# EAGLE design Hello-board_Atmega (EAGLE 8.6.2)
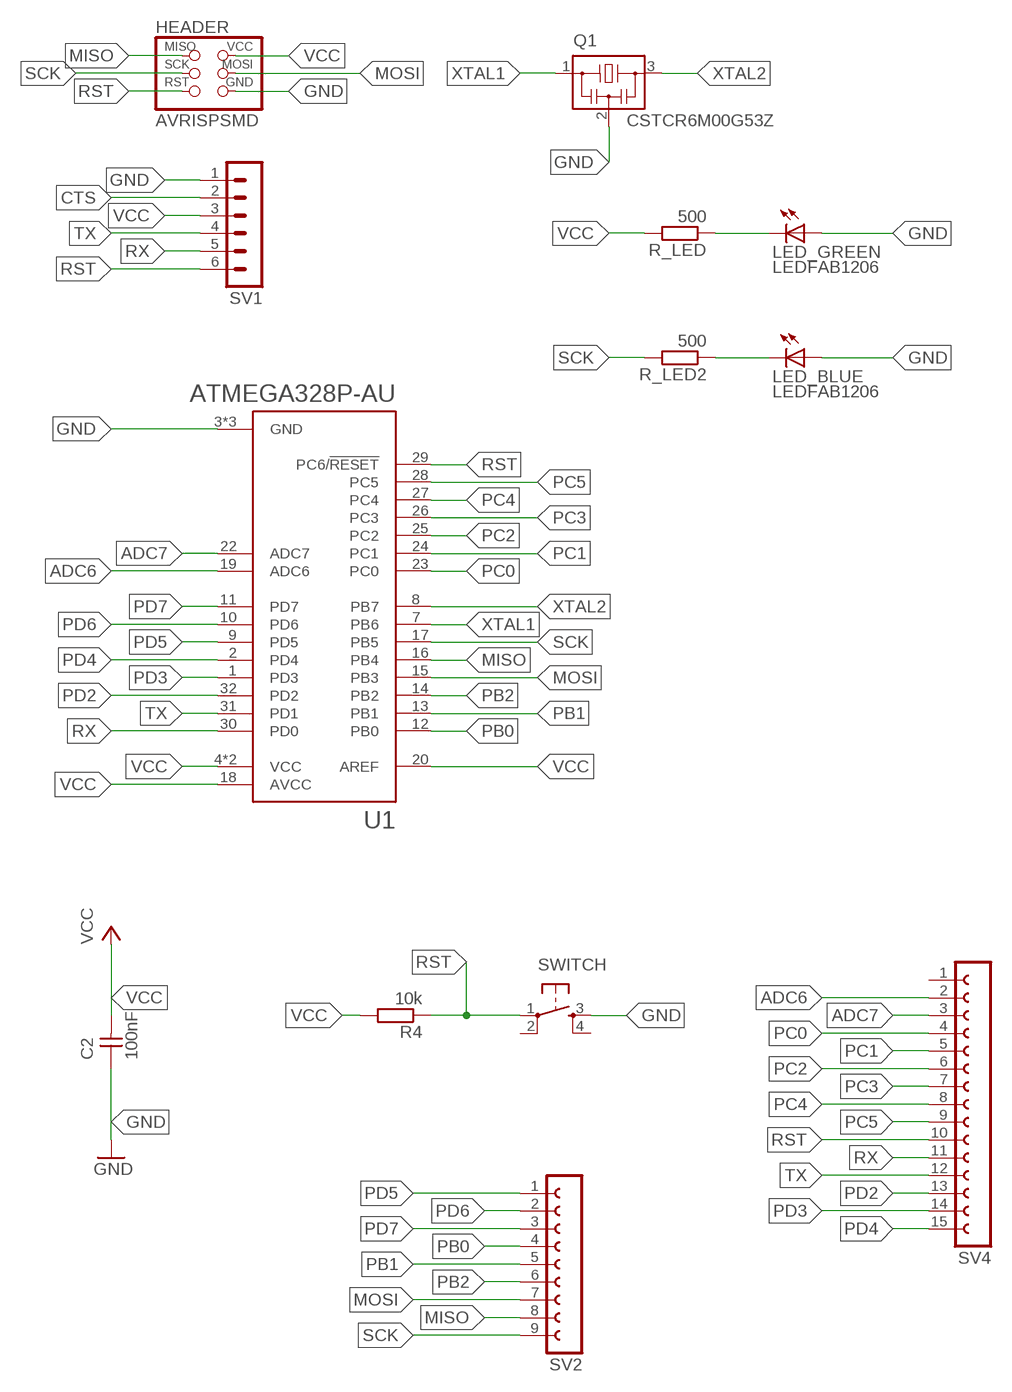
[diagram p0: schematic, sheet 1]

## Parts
C2  100nF  CAP-UNPOLARIZEDFAB  [C1206FAB]
HEADER  AVRISPSMD  [2X03SMD]
LED_BLUE  LEDFAB1206  [LED1206FAB]
LED_GREEN  LEDFAB1206  [LED1206FAB]
Q1  CSTCR6M00G53Z  [CSTCR6M]
R4  10k  R-EU_R1206  [R1206]
R_LED  500  R-EU_R1206  [R1206]
R_LED2  500  R-EU_R1206  [R1206]
SV1  MA06-1  [MA06-1]
SV2  FE09-1  [FE09]
SV4  FE15-1  [FE15]
SWITCH  6MM_SWITCH6MM_SWITCH  [6MM_SWITCH]
U1  ATMEGA328P-AU  [QFP80P900X900X120-32N]

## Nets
ADC6: SV4.2 U1.19(ADC6)
ADC7: SV4.3 U1.22(ADC7)
CTS: SV1.2
GND: C2.1 HEADER.6(GND) LED_BLUE.1(A) LED_GREEN.1(A) Q1.2 SV1.1 SWITCH.3(S) U1.3(GND) U1.5(GND) U1.21(GND)
MISO: HEADER.1(MISO) SV2.8 U1.16(PB4)
MOSI: HEADER.4(MOSI) SV2.7 U1.15(PB3)
N$21: LED_GREEN.2(C) R_LED.1
N$22: LED_BLUE.2(C) R_LED2.1
PB0: SV2.4 U1.12(PB0)
PB1: SV2.5 U1.13(PB1)
PB2: SV2.6 U1.14(PB2)
PC0: SV4.4 U1.23(PC0)
PC1: SV4.5 U1.24(PC1)
PC2: SV4.6 U1.25(PC2)
PC3: SV4.7 U1.26(PC3)
PC4: SV4.8 U1.27(PC4)
PC5: SV4.9 U1.28(PC5)
PD2: SV4.13 U1.32(PD2)
PD3: SV4.14 U1.1(PD3)
PD4: SV4.15 U1.2(PD4)
PD5: SV2.1 U1.9(PD5)
PD6: SV2.2 U1.10(PD6)
PD7: SV2.3 U1.11(PD7)
RST: HEADER.5(RST) R4.1 SV1.6 SV4.10 SWITCH.1(P) U1.29(PC6/!RESET)
RX: SV1.5 SV4.11 U1.30(PD0)
SCK: HEADER.3(SCK) R_LED2.2 U1.17(PB5)
TX: SV1.4 SV4.12 U1.31(PD1)
VCC: C2.2 HEADER.2(VCC) R4.2 R_LED.2 SV1.3 U1.4(VCC) U1.6(VCC) U1.18(AVCC) U1.20(AREF)
XTAL1: Q1.1 U1.7(PB6)
XTAL2: Q1.3 U1.8(PB7)
Unconnected: SV2.9 SV4.1 SWITCH.2(P1) SWITCH.4(S1)

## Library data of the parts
C2 = fab:CAP-UNPOLARIZED
HEADER = fab:AVRISP
LED_BLUE LED_GREEN = fab:LED: LED
Q1 = murata-filter:CSTCR: Resonator Source: murata.co.jp; MPN: CSTCR6M00G53-R0; OC_FARNELL: 1170434; OC_NEWARK: 25M8759
R4 R_LED R_LED2 = resistor:R-EU_: RESISTOR, European symbol
SV1 = con-lstb:MA06-1: PIN HEADER; OC_FARNELL: unknown; OC_NEWARK: unknown
SV2 = con-lsta:FE09-1: FEMALE HEADER; OC_FARNELL: unknown; OC_NEWARK: unknown
SV4 = con-lsta:FE15-1: FEMALE HEADER; OC_FARNELL: unknown; OC_NEWARK: unknown
SWITCH = fab:6MM_SWITCH: OMRON SWITCH
U1 = ATMEGA328P-AU:ATMEGA328P-AU: ATmega Series 20 MHz 32 KB Flash 2 KB SRAM 8-Bit Microcontroller - TQFP-32; AVAILABILITY: Good; DESCRIPTION: ATmega Series 20 MHz 32 KB Flash 2 KB SRAM 8-Bit Microcontroller - TQFP-32; MF: Atmel; MP: ATMEGA328P-AU; PACKAGE: TQFP-32 Atmel; PRICE: 2.38 USD

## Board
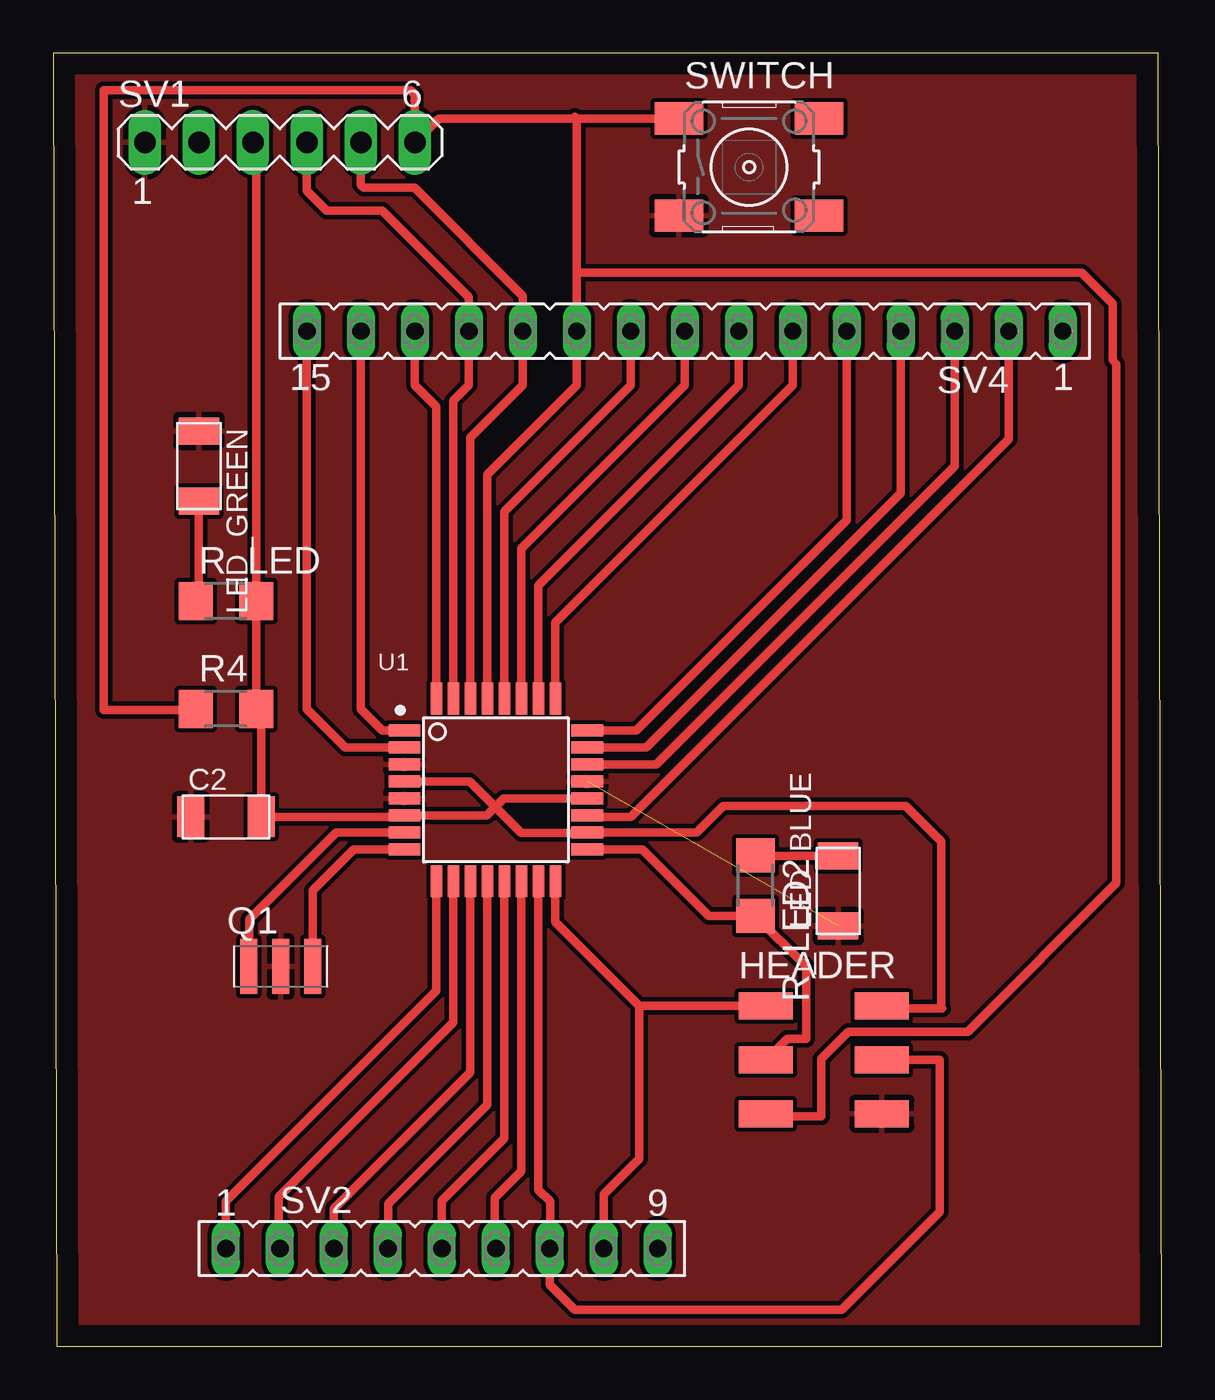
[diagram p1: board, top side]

Size 52.17 x 60.88 mm. Coordinates in mm from the lower left corner, seen from the top.
Outline: 0.17,0 52.17,0 52,60.88 0,60.88 0.17,0
Copper layers (1*16): Top 0.035mm / dielectric 1.5mm / Bottom 0.035mm
Design rules "default *": minimum track width 6mil, minimum drill 0.35mm, track to track 8mil, track to pad 8mil, pad to pad 8mil, via to via 8mil, smd to smd 8mil, copper to edge 40mil, drill to drill 8mil, minimum pad ring 10mil, minimum via ring 8mil, stop-mask expansion 4mil, vias tented up to drill 0mil, thermal gap 10mil

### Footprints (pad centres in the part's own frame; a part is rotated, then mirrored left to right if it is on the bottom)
C1206FAB = smd 1.27 x 1.905: 1 -1.651,0; 2 1.651,0
2X03SMD = smd 2.54 x 1.27: 1 -2.54,2.54; 2 2.92,2.54; 3 -2.54,0; 4 2.92,0; 5 -2.54,-2.54; 6 2.92,-2.54
LED1206FAB = smd 1.27 x 1.905: 1 -1.651,0; 2 1.651,0
CSTCR6M = smd 0.8 x 2.6: 1 -1.5,0; 2 0,0; 3 1.5,0
R1206 = smd 1.6 x 1.803: 1 -1.422,0; 2 1.422,0
MA06-1 = drill 1.016 long: 1 -6.35,0; 2 -3.81,0; 3 -1.27,0; 4 1.27,0; 5 3.81,0; 6 6.35,0
FE09 = drill 0.813 long: 1 -10.16,0; 2 -7.62,0; 3 -5.08,0; 4 -2.54,0; 5 0,0; 6 2.54,0; 7 5.08,0; 8 7.62,0; 9 10.16,0
FE15 = drill 0.813 long: 1 -17.78,0; 2 -15.24,0; 3 -12.7,0; 4 -10.16,0; 5 -7.62,0; 6 -5.08,0; 7 -2.54,0; 8 0,0; 9 2.54,0; 10 5.08,0; 11 7.62,0; 12 10.16,0; 13 12.7,0; 14 15.24,0; 15 17.78,0
6MM_SWITCH = smd 2.286 x 1.524: 1 -3.302,2.286; 2 3.302,2.286; 3 -3.302,-2.286; 4 3.302,-2.286
QFP80P900X900X120-32N = smd 1.5 x 0.55: 1 -4.3,2.8; 2 -4.3,2; 3 -4.3,1.2; 4 -4.3,0.4; 5 -4.3,-0.4; 6 -4.3,-1.2; 7 -4.3,-2; 8 -4.3,-2.8; 17 4.3,-2.8; 18 4.3,-2; 19 4.3,-1.2; 20 4.3,-0.4; 21 4.3,0.4; 22 4.3,1.2; 23 4.3,2; 24 4.3,2.8 | smd 0.55 x 1.5: 9 -2.8,-4.3; 10 -2,-4.3; 11 -1.2,-4.3; 12 -0.4,-4.3; 13 0.4,-4.3; 14 1.2,-4.3; 15 2,-4.3; 16 2.8,-4.3; 25 2.8,4.3; 26 2,4.3; 27 1.2,4.3; 28 0.4,4.3; 29 -0.4,4.3; 30 -1.2,4.3; 31 -2,4.3; 32 -2.8,4.3

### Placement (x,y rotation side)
C2  8.13,24.92 0 top
HEADER  36.07,13.49 0 top
LED_BLUE  36.94,21.44 90 top
LED_GREEN  6.86,41.43 270 top
Q1  10.71,17.89 0 top
R4  8.13,30 0 top
R_LED  8.13,35.08 0 top
R_LED2  33.05,21.69 270 top
SV1  10.67,56.67 0 top
SV2  18.29,4.6 0 top
SV4  29.72,47.78 180 top
SWITCH  32.74,55.51 0 top
U1  20.83,26.19 0 top

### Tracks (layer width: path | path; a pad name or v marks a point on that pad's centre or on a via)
ADC6
  Top 0.406: U1.19 25.2,24.92 27.18,24.92 44.96,42.7 SV4.2
ADC7
  Top 0.406: U1.22 28.38,27.39 42.42,41.43 SV4.3
GND  (1 unrouted)
  pour Top: -45.21,83.34 -45.21,-52.55 -43.94,-53.82 71.63,-53.82 77.98,-47.47 77.98,84.61 67.82,94.77 -33.78,94.77
MISO
  Top 0.406: U1.16 23.63,19.98 27.58,16.03 | 27.58,16.03 HEADER.1 | 27.58,16.03 27.58,8.83 25.91,7.16 SV2.8
MOSI
  Top 0.406: HEADER.4 39.01,13.48 41.72,13.48 41.72,6.34 37.1,1.72 24.55,1.72 23.37,2.89 SV2.7 23.38,6.82 22.83,7.37 U1.15
N$21
  Top 0.406: R_LED.1 6.86,35.24 LED_GREEN.2
N$22
  Top 0.406: R_LED2.1 33.07,23.09 LED_BLUE.2
PB0
  Top 0.406: U1.12 20.43,11.38 15.77,6.71 15.77,4.62 SV2.4
PB1
  Top 0.406: U1.13 21.23,9.8 18.29,6.86 SV2.5
PB2
  Top 0.406: U1.14 22.03,8.25 20.78,7 20.78,4.65 SV2.6
PC0
  Top 0.406: U1.23 27.91,28.19 39.88,40.16 SV4.4
PC1
  Top 0.406: U1.24 27.44,28.99 37.34,38.89 SV4.5
PC2
  Top 0.406: U1.25 23.63,34.07 34.8,45.24 SV4.6
PC3
  Top 0.406: U1.26 22.83,35.81 32.26,45.24 SV4.7
PC4
  Top 0.406: U1.27 22.03,37.55 29.72,45.24 SV4.8
PC5
  Top 0.406: U1.28 21.23,39.29 27.18,45.24 SV4.9
PD2
  Top 0.406: U1.32 18.03,44.23 17.02,45.24 SV4.13
PD3
  Top 0.406: U1.1 15.49,28.99 14.48,30 SV4.14
PD4
  Top 0.406: U1.2 13.75,28.19 11.94,30 SV4.15
PD5
  Top 0.406: U1.9 18.03,16.74 8.12,6.82 8.12,4.62 SV2.1
PD6
  Top 0.406: U1.10 18.83,15.26 10.61,7.03 10.61,4.67 SV2.2
PD7
  Top 0.406: U1.11 19.63,12.89 13.21,6.47 SV2.3
RST
  Top 0.406: U1.29 20.43,41.03 24.64,45.24 SV4.10 24.64,50.54 | 24.64,50.54 24.64,57.79 | 24.64,57.79 24.64,57.8 | 24.56,57.88 24.64,57.8 | 24.64,57.8 SWITCH.1 | 24.64,57.79 18.14,57.79 SV1.6 17.02,58.93 16.83,59.12 2.39,59.12 2.39,29.96 6.67,29.96 R4.1 | 24.64,50.54 48.4,50.54 49.86,49.08 49.86,46.41 50.03,46.23 50.03,21.81 43.03,14.8 37.42,14.8 36.15,13.53 36.15,10.83 33.65,10.83 HEADER.5
RX
  Top 0.406: U1.30 19.63,42.77 22.1,45.24 SV4.11 22.1,49.44 17.01,54.53 14.63,54.53 14.48,54.68 SV1.5
SCK
  Top 0.406: U1.17 27.73,23.39 30.86,20.27 R_LED2.2 35.43,17.88 35.43,14.47 34.53,14.47 33.55,13.48 HEADER.3
TX
  Top 0.406: U1.31 18.83,44.51 19.56,45.24 SV4.12 19.56,49.38 15.48,53.46 12.88,53.46 11.94,54.4 SV1.4
VCC
  Top 0.406: U1.4 19.6,26.59 20.81,25.39 | 20.81,25.39 22.02,24.17 25.11,24.17 U1.18 30.29,24.19 31.54,25.44 40.11,25.44 41.79,23.76 41.79,15.95 41.84,15.9 39.12,15.9 HEADER.2 | 20.81,25.39 20.41,24.99 U1.6 16.46,24.92 C2.2 9.78,29.78 R4.2 R_LED.2 9.55,56.52 SV1.3 | U1.20 21.21,25.79 20.81,25.39
XTAL1
  Top 0.406: U1.7 13.31,24.19 9.22,20.1 9.22,17.9 Q1.1
XTAL2
  Top 0.406: U1.8 14.15,23.39 12.21,21.45 Q1.3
